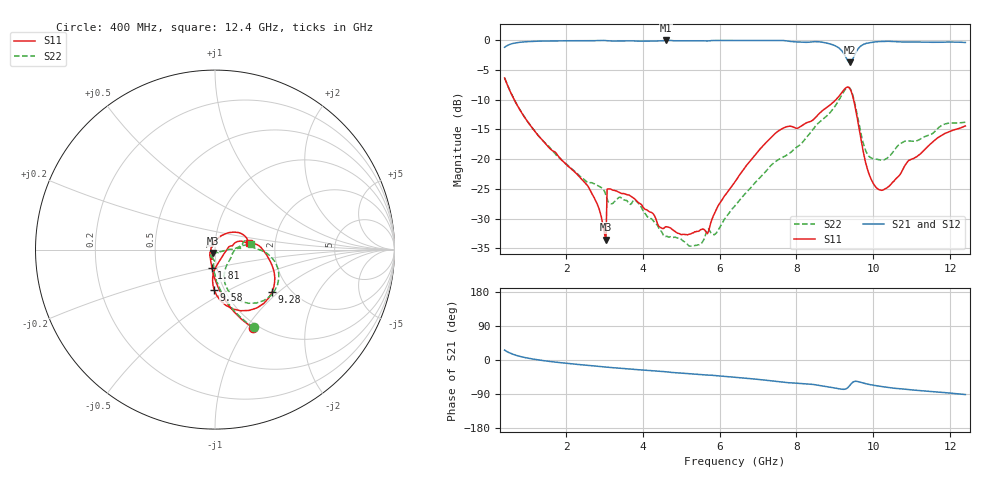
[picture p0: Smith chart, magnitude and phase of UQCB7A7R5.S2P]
!  Part Number  UQCB7A7R5  Mounting Orientation: Vertical
!  Description: RF capacitors
!  Application: Coupling, Bypass, Tuning, DC Block
!  Filters, Matching
# GHZ S DB R 50
! Freq  |S11|  S11 Ph  |S21|  S21 Ph  |S12|  S12 Ph  |S22|  S22 Ph
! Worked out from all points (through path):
!   401 points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, 400 MHz to 12.4 GHz, reference 50 ohm
!   highest |S21| = -0.01 dB at 4.6 GHz (marker M1); lowest = -3.7 dB at 9.4 GHz (marker M2)
!   group delay of S21, straight-line fit = 22.7 ps
!   lowest |S11| = -33.5 dB at 3.04 GHz (marker M3), VSWR 1.04, Z = 48.9 - j1.79 ohm
!   |S11| at or under -10 dB: 651.1 MHz to 9.027 GHz (8.375 GHz wide, 173 % of centre); 9.489 GHz to end of sweep
!   |S22| runs from -34.7 to -6.3 dB; largest |S21 - S12| = 0.0015
!   S11 on the Smith chart (normalised r, x): 400 MHz: 0.94, -1.07; 1.81 GHz: 0.94, -0.20; 9.28 GHz: 1.62, -0.91; 9.58 GHz: 0.90, -0.42; 12.4 GHz: 1.45, +0.11
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0.4  -6.33 -64.2  -1.16 26.1  -1.15 26.1  -6.31 -63.6
0.85  -12.24 -82.2  -0.28 8.3  -0.28 8.3  -12.23 -81.0
1.81  -19.60 -99.8  -0.08 -6.5  -0.08 -6.5  -19.68 -93.7
2.41  -23.39 -110.5  -0.05 -12.7  -0.05 -12.7  -23.12 -95.3
2.98  -31.79 -126.5  -0.01 -18.1  -0.01 -18.1  -25.17 -99.9
3.04  -33.54 -119.5  -0.03 -18.8  -0.02 -18.8  -26.16 -104.1
3.13  -25.01 -107.0  -0.08 -19.7  -0.08 -19.7  -27.42 -110.3
3.82  -26.89 -129.6  -0.11 -25.4  -0.11 -25.4  -27.04 -121.2
4.42  -31.35 -150.6  -0.08 -29.5  -0.08 -29.5  -31.68 -125.2
4.6  -31.38 -150.5  -0.01 -31.0  -0.01 -31.0  -33.03 -113.6
5.29  -32.44 154.6  -0.06 -36.8  -0.06 -36.9  -34.63 -77.8
5.68  -32.57 115.5  -0.10 -39.6  -0.09 -39.6  -31.80 -48.0
6.4  -23.84 76.2  -0.01 -45.6  -0.01 -45.7  -27.85 -13.6
7.48  -15.50 33.2  -0.01 -56.7  -0.01 -56.7  -20.30 0.6
8.41  -13.50 8.8  -0.23 -64.1  -0.23 -64.1  -15.19 8.3
8.98  -10.30 -10.0  -0.82 -73.5  -0.82 -73.6  -11.32 -2.3
9.28  -8.03 -36.7  -2.75 -76.6  -2.75 -76.6  -8.18 -24.3
9.4  -8.21 -60.7  -3.72 -65.8  -3.72 -65.8  -8.12 -46.5
9.58  -12.96 -91.1  -1.67 -56.5  -1.67 -56.5  -12.44 -72.2
9.97  -23.70 -64.6  -0.32 -66.0  -0.33 -66.0  -19.87 -39.7
10.42  -24.52 -10.4  -0.16 -72.9  -0.16 -73.0  -19.53 -4.9
12.4  -14.42 10.9  -0.34 -91.2  -0.34 -91.2  -13.78 8.8
